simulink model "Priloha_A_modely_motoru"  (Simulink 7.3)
settings: Solver=ode23tb  StartTime=0.0  StopTime=0.5  RelTol=1e-3
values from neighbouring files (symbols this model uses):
  ILi = [0 Imax]    [Priloha_B_motor1_parametry.m]    (also in Priloha_C_motor2_parametry.m)
  Im = Psim / Ldi(1)    [Priloha_B_motor1_parametry.m]    (also in Priloha_C_motor2_parametry.m)
  Imax = 8    [Priloha_B_motor1_parametry.m]    (also in Priloha_C_motor2_parametry.m)
  J = 7e-3    (= 0.007)    [Priloha_B_motor1_parametry.m]    (also in Priloha_C_motor2_parametry.m)
  Ld = 22.5e-3    (= 0.0225)    [Priloha_B_motor1_parametry.m]    (also in Priloha_C_motor2_parametry.m)
  Ldi = [Ldi Ldi]    [Priloha_B_motor1_parametry.m]    (also in Priloha_C_motor2_parametry.m)
  Lq = 54e-3    (= 0.054)    [Priloha_B_motor1_parametry.m]    (also in Priloha_C_motor2_parametry.m)
  Lqi = [Lqi Lqi]    [Priloha_B_motor1_parametry.m]    (also in Priloha_C_motor2_parametry.m)
  p = 3    [Priloha_B_motor1_parametry.m]    (also in Priloha_C_motor2_parametry.m)
  Psim = 238.2e-3    (= 0.2382)    [Priloha_B_motor1_parametry.m]    (also in Priloha_C_motor2_parametry.m = 0.181)
  Rs = 3.95    [Priloha_B_motor1_parametry.m]    (also in Priloha_C_motor2_parametry.m)

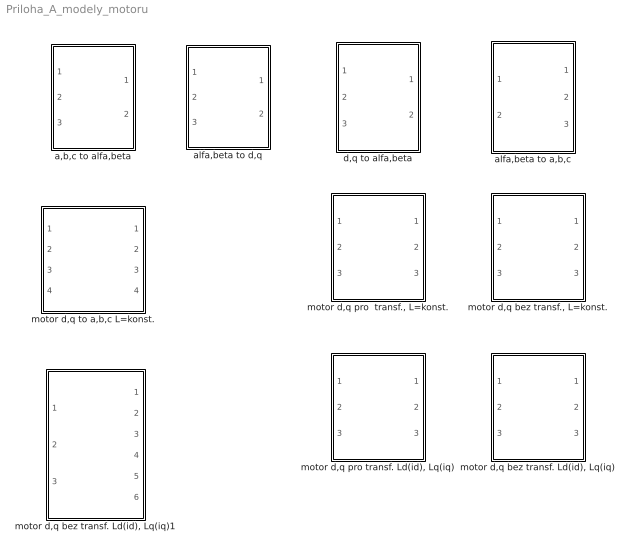
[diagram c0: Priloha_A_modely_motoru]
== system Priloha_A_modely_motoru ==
  a,b,c to alfa,beta : Subsystem
  alfa,beta to a,b,c : Subsystem
  alfa,beta to d,q : Subsystem
  d,q to alfa,beta : Subsystem
  "motor d,q bez transf., L=konst." : Subsystem
  "motor d,q bez transf. Ld(id), Lq(iq)" : Subsystem
  "motor d,q bez transf. Ld(id), Lq(iq)1" : Subsystem
  "motor d,q pro  transf., L=konst." : Subsystem
  "motor d,q pro transf. Ld(id), Lq(iq)" : Subsystem
  motor d,q to a,b,c L=konst. : Subsystem

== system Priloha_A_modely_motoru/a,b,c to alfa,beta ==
  note: transformace a, b, c do alfa, beta
  a : Inport  OutDataType=fixdt(1, 16)  OutScaling=2^0
  b : Inport  Port=2  OutDataType=fixdt(1, 16)  OutScaling=2^0
  c : Inport  Port=3  OutDataType=fixdt(1, 16)  OutScaling=2^0
  Add3 : Sum  Inputs=+-  OutDataType=fixdt(1, 16)  OutScaling=2^-10
  Gain6 : Gain  Gain=1/(sqrt(3))  ParameterDataType=fixdt(1, 16)  ParameterScaling=2^0  OutDataType=fixdt(1, 16)  OutScaling=2^0
  alfa : Outport  OutDataType=fixdt(1, 16)  OutScaling=2^0
  beta : Outport  Port=2  OutDataType=fixdt(1, 16)  OutScaling=2^0
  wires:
  a/1 -> alfa/1
  Gain6/1 -> beta/1
  Add3/1 -> Gain6/1
  b/1 -> Add3/1
  c/1 -> Add3/2

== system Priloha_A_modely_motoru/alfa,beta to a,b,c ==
  note: transformace alfa, beta do a, b, c
  alfa : Inport  OutDataType=fixdt(1, 16)  OutScaling=2^0
  beta : Inport  Port=2  OutDataType=fixdt(1, 16)  OutScaling=2^0
  Add1 : Sum  Inputs=--  OutDataType=fixdt(1, 16)  OutScaling=2^-10
  Add5 : Sum  Inputs=-+  OutDataType=fixdt(1, 16)  OutScaling=2^-10
  Gain1 : Gain  Gain=1/2  ParameterDataType=fixdt(1, 16)  ParameterScaling=2^0  OutDataType=fixdt(1, 16)  OutScaling=2^0
  Gain2 : Gain  Gain=sqrt(3)/2  ParameterDataType=fixdt(1, 16)  ParameterScaling=2^0  OutDataType=fixdt(1, 16)  OutScaling=2^0
  a : Outport  OutDataType=fixdt(1, 16)  OutScaling=2^0
  b : Outport  Port=2  OutDataType=fixdt(1, 16)  OutScaling=2^0
  c : Outport  Port=3  OutDataType=fixdt(1, 16)  OutScaling=2^0
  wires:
  alfa/1 -> a/1, Gain1/1
  Gain1/1 -> Add5/1, Add1/1
  Add5/1 -> b/1
  beta/1 -> Gain2/1
  Add1/1 -> c/1
  Gain2/1 -> Add5/2, Add1/2

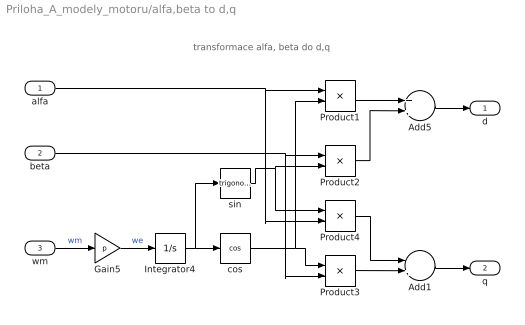
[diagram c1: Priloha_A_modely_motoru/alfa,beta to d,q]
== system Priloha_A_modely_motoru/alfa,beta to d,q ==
  note: transformace alfa, beta do d,q
  alfa : Inport  OutDataType=fixdt(1, 16)  OutScaling=2^0
  beta : Inport  Port=2  OutDataType=fixdt(1, 16)  OutScaling=2^0
  wm : Inport  Port=3  OutDataType=fixdt(1, 16)  OutScaling=2^0
  Add1 : Sum  Inputs=-+  OutDataType=fixdt(1, 16)  OutScaling=2^-10
  Add5 : Sum  OutDataType=fixdt(1, 16)  OutScaling=2^-10
  Gain5 : Gain  Gain=p  ParameterDataType=fixdt(1, 16)  ParameterScaling=2^0  OutDataType=fixdt(1, 16)  OutScaling=2^0
  Integrator4 : Integrator
  Product{1..4} (4 alike) : Product  OutDataType=fixdt(1, 16)  OutScaling=2^0
  cos : Trigonometry  Operator=cos  OutputSignalType=real
  sin : Trigonometry  OutputSignalType=real
  d : Outport  OutDataType=fixdt(1, 16)  OutScaling=2^0
  q : Outport  Port=2  OutDataType=fixdt(1, 16)  OutScaling=2^0
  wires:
  cos/1 -> Product1/2, Product3/1
  sin/1 -> Product4/1, Product2/2
  Integrator4/1 -> sin/1, cos/1
  Gain5/1 -> Integrator4/1  "we"
  wm/1 -> Gain5/1  "wm"
  Add1/1 -> q/1
  Product2/1 -> Add5/2
  beta/1 -> Product3/2, Product2/1
  alfa/1 -> Product4/2, Product1/1
  Product1/1 -> Add5/1
  Add5/1 -> d/1
  Product4/1 -> Add1/1
  Product3/1 -> Add1/2

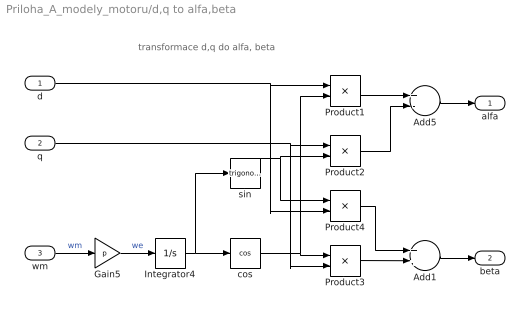
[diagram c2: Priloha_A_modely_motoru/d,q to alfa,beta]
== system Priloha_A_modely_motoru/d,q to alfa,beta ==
  note: transformace d,q do alfa, beta
  d : Inport  OutDataType=fixdt(1, 16)  OutScaling=2^0
  q : Inport  Port=2  OutDataType=fixdt(1, 16)  OutScaling=2^0
  wm : Inport  Port=3  OutDataType=fixdt(1, 16)  OutScaling=2^0
  Add1 : Sum  OutDataType=fixdt(1, 16)  OutScaling=2^-10
  Add5 : Sum  Inputs=+-  OutDataType=fixdt(1, 16)  OutScaling=2^-10
  Gain5 : Gain  Gain=p  ParameterDataType=fixdt(1, 16)  ParameterScaling=2^0  OutDataType=fixdt(1, 16)  OutScaling=2^0
  Integrator4 : Integrator
  Product{1..4} (4 alike) : Product  OutDataType=fixdt(1, 16)  OutScaling=2^0
  cos : Trigonometry  Operator=cos
  sin : Trigonometry
  alfa : Outport  OutDataType=fixdt(1, 16)  OutScaling=2^0
  beta : Outport  Port=2  OutDataType=fixdt(1, 16)  OutScaling=2^0
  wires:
  Add5/1 -> alfa/1
  Product1/1 -> Add5/1
  d/1 -> Product4/2, Product1/1
  q/1 -> Product3/2, Product2/1
  Product2/1 -> Add5/2
  Add1/1 -> beta/1
  wm/1 -> Gain5/1  "wm"
  Gain5/1 -> Integrator4/1  "we"
  Integrator4/1 -> sin/1, cos/1
  sin/1 -> Product4/1, Product2/2
  cos/1 -> Product1/2, Product3/1
  Product4/1 -> Add1/1
  Product3/1 -> Add1/2

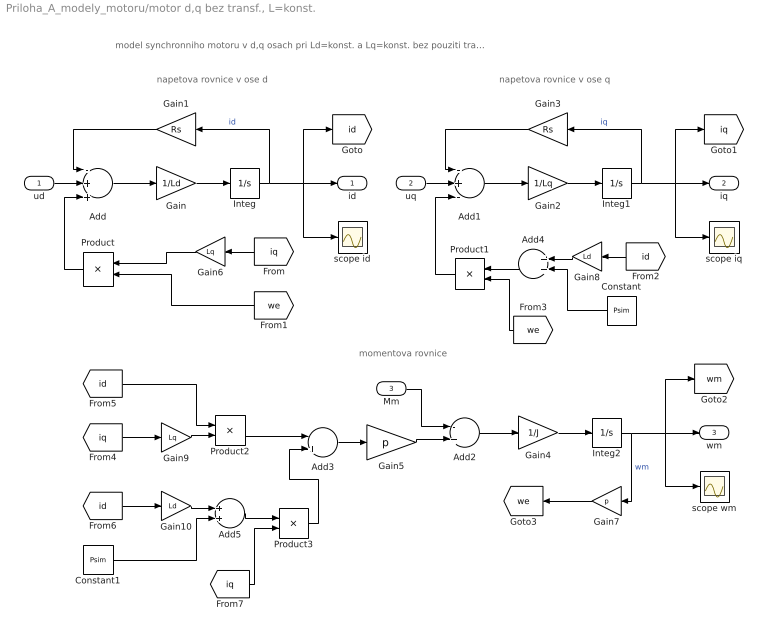
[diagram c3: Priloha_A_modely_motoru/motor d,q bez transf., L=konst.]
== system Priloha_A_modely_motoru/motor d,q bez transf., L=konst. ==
  note: momentova rovnice
  note: napetova rovnice v ose q
  note: napetova rovnice v ose d
  note: model synchronniho motoru v d,q osach pri Ld=konst. a Lq=konst. bez pouziti transformace (v momentove rovnici neni koeficient 3/2)
  ud : Inport  OutDataType=fixdt(1, 16)  OutScaling=2^0
  uq : Inport  Port=2  OutDataType=fixdt(1, 16)  OutScaling=2^0
  Mm : Inport  Port=3  OutDataType=fixdt(1, 16)  OutScaling=2^0
  Add : Sum  Inputs=-++  OutDataType=fixdt(1, 16)  OutScaling=2^-10
  Add1 : Sum  Inputs=-+-  OutDataType=fixdt(1, 16)  OutScaling=2^-10
  Add2 : Sum  Inputs=-+  OutDataType=fixdt(1, 16)  OutScaling=2^-10
  Add3 : Sum  Inputs=-+  OutDataType=fixdt(1, 16)  OutScaling=2^-10
  Add4 : Sum  OutDataType=fixdt(1, 16)  OutScaling=2^-10
  Add5 : Sum  OutDataType=fixdt(1, 16)  OutScaling=2^-10
  Constant : Constant  Value=Psim  OutDataType=fixdt(1, 16)  OutScaling=2^0
  Constant1 : Constant  Value=Psim  OutDataType=fixdt(1, 16)  OutScaling=2^0
  Gain : Gain  Gain=1/Ld  ParameterDataType=fixdt(1, 16)  ParameterScaling=2^0  OutDataType=fixdt(1, 16)  OutScaling=2^0
  Gain1 : Gain  Gain=Rs  ParameterDataType=fixdt(1, 16)  ParameterScaling=2^0  OutDataType=fixdt(1, 16)  OutScaling=2^0
  Gain10 : Gain  Gain=Ld  ParameterDataType=fixdt(1, 16)  ParameterScaling=2^0  OutDataType=fixdt(1, 16)  OutScaling=2^0
  Gain2 : Gain  Gain=1/Lq  ParameterDataType=fixdt(1, 16)  ParameterScaling=2^0  OutDataType=fixdt(1, 16)  OutScaling=2^0
  Gain3 : Gain  Gain=Rs  ParameterDataType=fixdt(1, 16)  ParameterScaling=2^0  OutDataType=fixdt(1, 16)  OutScaling=2^0
  Gain4 : Gain  Gain=1/J  ParameterDataType=fixdt(1, 16)  ParameterScaling=2^0  OutDataType=fixdt(1, 16)  OutScaling=2^0
  Gain5 : Gain  Gain=p  ParameterDataType=fixdt(1, 16)  ParameterScaling=2^0  OutDataType=fixdt(1, 16)  OutScaling=2^0
  Gain6 : Gain  Gain=Lq  ParameterDataType=fixdt(1, 16)  ParameterScaling=2^0  OutDataType=fixdt(1, 16)  OutScaling=2^0
  Gain7 : Gain  Gain=p  ParameterDataType=fixdt(1, 16)  ParameterScaling=2^0  OutDataType=fixdt(1, 16)  OutScaling=2^0
  Gain8 : Gain  Gain=Ld  ParameterDataType=fixdt(1, 16)  ParameterScaling=2^0  OutDataType=fixdt(1, 16)  OutScaling=2^0
  Gain9 : Gain  Gain=Lq  ParameterDataType=fixdt(1, 16)  ParameterScaling=2^0  OutDataType=fixdt(1, 16)  OutScaling=2^0
  Integ : Integrator
  Integ1 : Integrator
  Integ2 : Integrator
  Product{,1..3} (4 alike) : Product  OutDataType=fixdt(1, 16)  OutScaling=2^0
  scope id : Scope
  scope iq : Scope
  scope wm : Scope
  id : Outport  OutDataType=fixdt(1, 16)  OutScaling=2^0
  iq : Outport  Port=2  OutDataType=fixdt(1, 16)  OutScaling=2^0
  wm : Outport  Port=3  OutDataType=fixdt(1, 16)  OutScaling=2^0
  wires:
  [we] -> Product/2
  Gain6/1 -> Product/1
  [iq] -> Gain6/1
  Constant/1 -> Add4/2
  Product/1 -> Add/3
  [we] -> Product1/2
  Product1/1 -> Add1/3
  Product3/1 -> Add3/2
  [iq] -> Product3/2
  Constant1/1 -> Add5/2
  Add5/1 -> Product3/1
  Gain10/1 -> Add5/1
  [id] -> Gain10/1
  Product2/1 -> Add3/1
  Gain9/1 -> Product2/2
  [id] -> Product2/1
  [iq] -> Gain9/1
  Add4/1 -> Product1/1
  Gain8/1 -> Add4/1
  [id] -> Gain8/1
  Gain7/1 -> [we]
  Add3/1 -> Gain5/1
  Mm/1 -> Add2/1
  Gain5/1 -> Add2/2
  Add2/1 -> Gain4/1
  Gain4/1 -> Integ2/1
  Integ2/1 -> Gain7/1, [wm], scope wm/1, wm/1  "wm"
  uq/1 -> Add1/2
  Gain3/1 -> Add1/1
  Add1/1 -> Gain2/1
  Gain2/1 -> Integ1/1
  Integ1/1 -> [iq], iq/1, scope iq/1, Gain3/1  "iq"
  ud/1 -> Add/2
  Gain1/1 -> Add/1
  Add/1 -> Gain/1
  Gain/1 -> Integ/1
  Integ/1 -> Gain1/1, [id], scope id/1, id/1  "id"

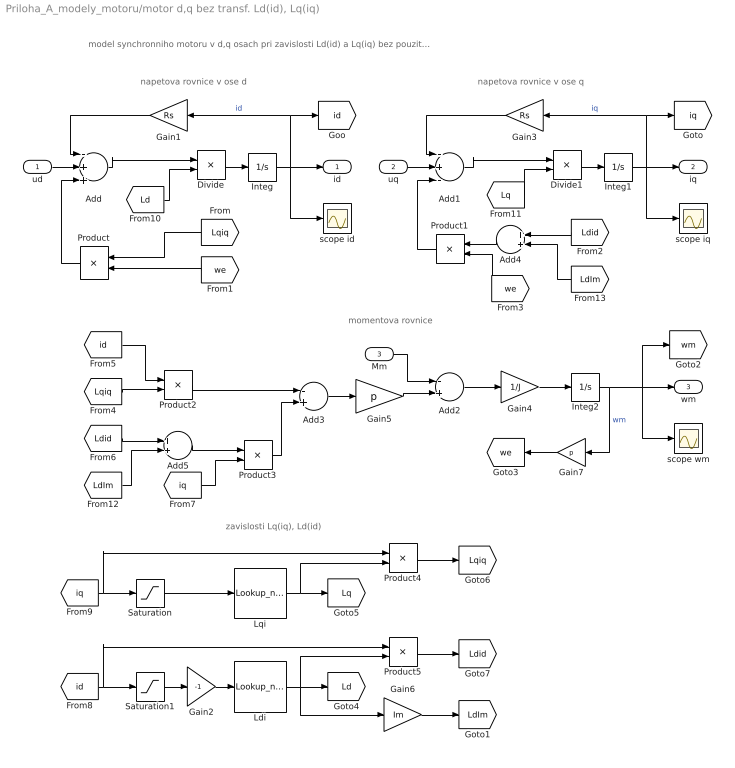
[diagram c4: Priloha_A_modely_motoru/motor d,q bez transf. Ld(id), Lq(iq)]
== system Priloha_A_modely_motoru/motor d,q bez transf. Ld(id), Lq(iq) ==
  note: zavislosti Lq(iq), Ld(id)
  note: momentova rovnice
  note: napetova rovnice v ose q
  note: napetova rovnice v ose d
  note: model synchronniho motoru v d,q osach pri zavislosti Ld(id) a Lq(iq) bez pouziti transformace (v momentove rovnici neni koeficient 3/2)
  ud : Inport  OutDataType=fixdt(1, 16)  OutScaling=2^0
  uq : Inport  Port=2  OutDataType=fixdt(1, 16)  OutScaling=2^0
  Mm : Inport  Port=3  OutDataType=fixdt(1, 16)  OutScaling=2^0
  Add : Sum  Inputs=-++  OutDataType=fixdt(1, 16)  OutScaling=2^-10
  Add1 : Sum  Inputs=-+-  OutDataType=fixdt(1, 16)  OutScaling=2^-10
  Add2 : Sum  Inputs=-+  OutDataType=fixdt(1, 16)  OutScaling=2^-10
  Add3 : Sum  Inputs=-+  OutDataType=fixdt(1, 16)  OutScaling=2^-10
  Add4 : Sum  OutDataType=fixdt(1, 16)  OutScaling=2^-10
  Add5 : Sum  OutDataType=fixdt(1, 16)  OutScaling=2^-10
  Divide : Product  Inputs=*/  OutDataType=fixdt(1, 16)  OutScaling=2^-10
  Divide1 : Product  Inputs=*/  OutDataType=fixdt(1, 16)  OutScaling=2^-10
  Gain1 : Gain  Gain=Rs  ParameterDataType=fixdt(1, 16)  ParameterScaling=2^0  OutDataType=fixdt(1, 16)  OutScaling=2^0
  Gain2 : Gain  Gain=-1  ParameterDataType=fixdt(1, 16)  ParameterScaling=2^0  OutDataType=fixdt(1, 16)  OutScaling=2^0
  Gain3 : Gain  Gain=Rs  ParameterDataType=fixdt(1, 16)  ParameterScaling=2^0  OutDataType=fixdt(1, 16)  OutScaling=2^0
  Gain4 : Gain  Gain=1/J  ParameterDataType=fixdt(1, 16)  ParameterScaling=2^0  OutDataType=fixdt(1, 16)  OutScaling=2^0
  Gain5 : Gain  Gain=p  ParameterDataType=fixdt(1, 16)  ParameterScaling=2^0  OutDataType=fixdt(1, 16)  OutScaling=2^0
  Gain6 : Gain  Gain=Im  ParameterDataType=fixdt(1, 16)  ParameterScaling=2^0  OutDataType=fixdt(1, 16)  OutScaling=2^0
  Gain7 : Gain  Gain=p  ParameterDataType=fixdt(1, 16)  ParameterScaling=2^0  OutDataType=fixdt(1, 16)  OutScaling=2^0
  Integ : Integrator
  Integ1 : Integrator
  Integ2 : Integrator
  Ldi : Lookup_n-D  NumberOfTableDimensions=1  BreakpointsForDimension1=[ILi]  Table=[Ldi]
  Lqi : Lookup_n-D  NumberOfTableDimensions=1  BreakpointsForDimension1=[ILi]  Table=[Lqi]
  Product{,1..5} (6 alike) : Product  OutDataType=fixdt(1, 16)  OutScaling=2^0
  Saturation : Saturate  UpperLimit=Imax  LowerLimit=ILi(1)  OutDataType=fixdt(1, 16)  OutScaling=2^0
  Saturation1 : Saturate  UpperLimit=ILi(1)  LowerLimit=-Imax  OutDataType=fixdt(1, 16)  OutScaling=2^0
  scope id : Scope
  scope iq : Scope
  scope wm : Scope
  id : Outport  OutDataType=fixdt(1, 16)  OutScaling=2^0
  iq : Outport  Port=2  OutDataType=fixdt(1, 16)  OutScaling=2^0
  wm : Outport  Port=3  OutDataType=fixdt(1, 16)  OutScaling=2^0
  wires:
  [LdIm] -> Add4/2
  [LdIm] -> Add5/2
  Gain6/1 -> [LdIm]
  Gain2/1 -> Ldi/1
  [Lq] -> Divide1/2
  Add1/1 -> Divide1/1
  [Lqiq] -> Product/1
  Divide1/1 -> Integ1/1
  [Ld] -> Divide/2
  Add/1 -> Divide/1
  Divide/1 -> Integ/1
  Product5/1 -> [Ldid]
  Product4/1 -> [Lqiq]
  Ldi/1 -> Gain6/1, Product5/2, [Ld]
  [id] -> Product5/1, Saturation1/1
  Lqi/1 -> Product4/2, [Lq]
  [iq] -> Product4/1, Saturation/1
  Saturation1/1 -> Gain2/1
  Saturation/1 -> Lqi/1
  [we] -> Product/2
  Product/1 -> Add/3
  [we] -> Product1/2
  Product1/1 -> Add1/3
  Product3/1 -> Add3/2
  [iq] -> Product3/2
  Add5/1 -> Product3/1
  [Ldid] -> Add5/1
  Product2/1 -> Add3/1
  [id] -> Product2/1
  [Lqiq] -> Product2/2
  Add4/1 -> Product1/1
  [Ldid] -> Add4/1
  Gain7/1 -> [we]
  Add3/1 -> Gain5/1
  Mm/1 -> Add2/1
  Gain5/1 -> Add2/2
  Add2/1 -> Gain4/1
  Gain4/1 -> Integ2/1
  Integ2/1 -> Gain7/1, [wm], scope wm/1, wm/1  "wm"
  uq/1 -> Add1/2
  Gain3/1 -> Add1/1
  Integ1/1 -> Gain3/1, [iq], iq/1, scope iq/1  "iq"
  ud/1 -> Add/2
  Gain1/1 -> Add/1
  Integ/1 -> Gain1/1, [id], scope id/1, id/1  "id"

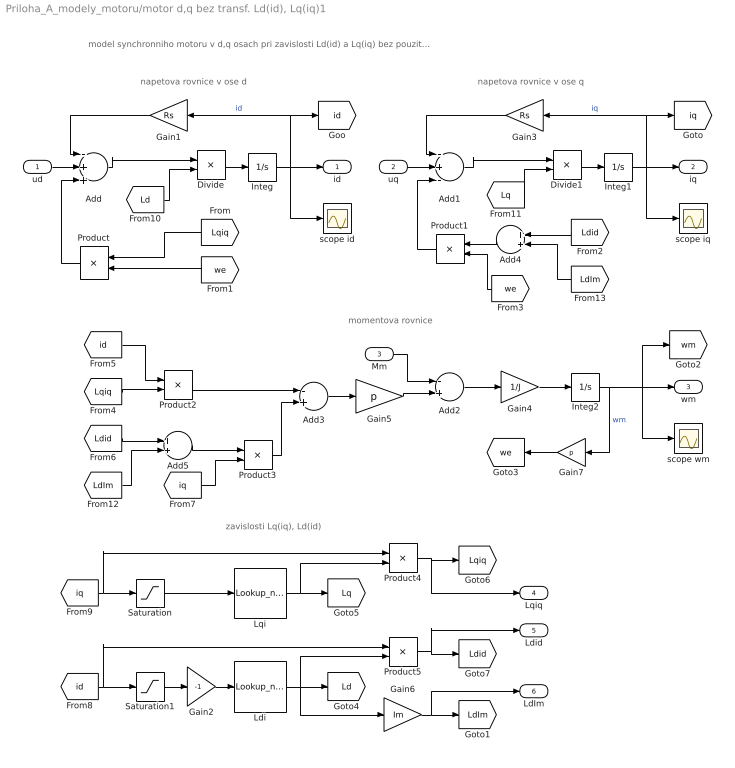
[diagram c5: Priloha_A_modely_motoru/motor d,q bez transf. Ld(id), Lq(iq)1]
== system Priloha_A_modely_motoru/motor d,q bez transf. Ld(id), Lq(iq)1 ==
  note: model synchronniho motoru v d,q osach pri zavislosti Ld(id) a Lq(iq) bez pouziti transformace (v momentove rovnici neni koeficient 3/2)
  note: napetova rovnice v ose d
  note: napetova rovnice v ose q
  note: momentova rovnice
  note: zavislosti Lq(iq), Ld(id)
  ud : Inport  OutDataType=fixdt(1, 16)  OutScaling=2^0
  uq : Inport  Port=2  OutDataType=fixdt(1, 16)  OutScaling=2^0
  Mm : Inport  Port=3  OutDataType=fixdt(1, 16)  OutScaling=2^0
  Add : Sum  Inputs=-++  OutDataType=fixdt(1, 16)  OutScaling=2^-10
  Add1 : Sum  Inputs=-+-  OutDataType=fixdt(1, 16)  OutScaling=2^-10
  Add2 : Sum  Inputs=-+  OutDataType=fixdt(1, 16)  OutScaling=2^-10
  Add3 : Sum  Inputs=-+  OutDataType=fixdt(1, 16)  OutScaling=2^-10
  Add4 : Sum  OutDataType=fixdt(1, 16)  OutScaling=2^-10
  Add5 : Sum  OutDataType=fixdt(1, 16)  OutScaling=2^-10
  Divide : Product  Inputs=*/  OutDataType=fixdt(1, 16)  OutScaling=2^-10
  Divide1 : Product  Inputs=*/  OutDataType=fixdt(1, 16)  OutScaling=2^-10
  Gain1 : Gain  Gain=Rs  ParameterDataType=fixdt(1, 16)  ParameterScaling=2^0  OutDataType=fixdt(1, 16)  OutScaling=2^0
  Gain2 : Gain  Gain=-1  ParameterDataType=fixdt(1, 16)  ParameterScaling=2^0  OutDataType=fixdt(1, 16)  OutScaling=2^0
  Gain3 : Gain  Gain=Rs  ParameterDataType=fixdt(1, 16)  ParameterScaling=2^0  OutDataType=fixdt(1, 16)  OutScaling=2^0
  Gain4 : Gain  Gain=1/J  ParameterDataType=fixdt(1, 16)  ParameterScaling=2^0  OutDataType=fixdt(1, 16)  OutScaling=2^0
  Gain5 : Gain  Gain=p  ParameterDataType=fixdt(1, 16)  ParameterScaling=2^0  OutDataType=fixdt(1, 16)  OutScaling=2^0
  Gain6 : Gain  Gain=Im  ParameterDataType=fixdt(1, 16)  ParameterScaling=2^0  OutDataType=fixdt(1, 16)  OutScaling=2^0
  Gain7 : Gain  Gain=p  ParameterDataType=fixdt(1, 16)  ParameterScaling=2^0  OutDataType=fixdt(1, 16)  OutScaling=2^0
  Integ : Integrator
  Integ1 : Integrator
  Integ2 : Integrator
  Ldi : Lookup_n-D  NumberOfTableDimensions=1  BreakpointsForDimension1=[ILi]  Table=[Ldi]
  Lqi : Lookup_n-D  NumberOfTableDimensions=1  BreakpointsForDimension1=[ILi]  Table=[Lqi]
  Product{,1..5} (6 alike) : Product  OutDataType=fixdt(1, 16)  OutScaling=2^0
  Saturation : Saturate  UpperLimit=Imax  LowerLimit=ILi(1)  OutDataType=fixdt(1, 16)  OutScaling=2^0
  Saturation1 : Saturate  UpperLimit=ILi(1)  LowerLimit=-Imax  OutDataType=fixdt(1, 16)  OutScaling=2^0
  scope id : Scope
  scope iq : Scope
  scope wm : Scope
  id : Outport  OutDataType=fixdt(1, 16)  OutScaling=2^0
  iq : Outport  Port=2  OutDataType=fixdt(1, 16)  OutScaling=2^0
  wm : Outport  Port=3  OutDataType=fixdt(1, 16)  OutScaling=2^0
  Lqiq : Outport  Port=4  OutDataType=fixdt(1, 16)  OutScaling=2^0
  Ldid : Outport  Port=5  OutDataType=fixdt(1, 16)  OutScaling=2^0
  LdIm : Outport  Port=6  OutDataType=fixdt(1, 16)  OutScaling=2^0
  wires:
  Integ/1 -> id/1, scope id/1, [id], Gain1/1  "id"
  Gain1/1 -> Add/1
  ud/1 -> Add/2
  Integ1/1 -> scope iq/1, iq/1, [iq], Gain3/1  "iq"
  Gain3/1 -> Add1/1
  uq/1 -> Add1/2
  Integ2/1 -> wm/1, scope wm/1, [wm], Gain7/1  "wm"
  Gain4/1 -> Integ2/1
  Add2/1 -> Gain4/1
  Gain5/1 -> Add2/2
  Mm/1 -> Add2/1
  Add3/1 -> Gain5/1
  Gain7/1 -> [we]
  [Ldid] -> Add4/1
  Add4/1 -> Product1/1
  [Lqiq] -> Product2/2
  [id] -> Product2/1
  Product2/1 -> Add3/1
  [Ldid] -> Add5/1
  Add5/1 -> Product3/1
  [iq] -> Product3/2
  Product3/1 -> Add3/2
  Product1/1 -> Add1/3
  Product/1 -> Add/3
  Saturation/1 -> Lqi/1
  Saturation1/1 -> Gain2/1
  [iq] -> Saturation/1, Product4/1
  Lqi/1 -> [Lq], Product4/2
  [id] -> Saturation1/1, Product5/1
  Ldi/1 -> [Ld], Product5/2, Gain6/1
  Product4/1 -> [Lqiq], Lqiq/1
  Product5/1 -> [Ldid], Ldid/1
  Divide/1 -> Integ/1
  Add/1 -> Divide/1
  [Ld] -> Divide/2
  Divide1/1 -> Integ1/1
  [Lqiq] -> Product/1
  Add1/1 -> Divide1/1
  [Lq] -> Divide1/2
  Gain2/1 -> Ldi/1
  Gain6/1 -> [LdIm], LdIm/1
  [LdIm] -> Add5/2
  [LdIm] -> Add4/2
  [we] -> Product1/2
  [we] -> Product/2

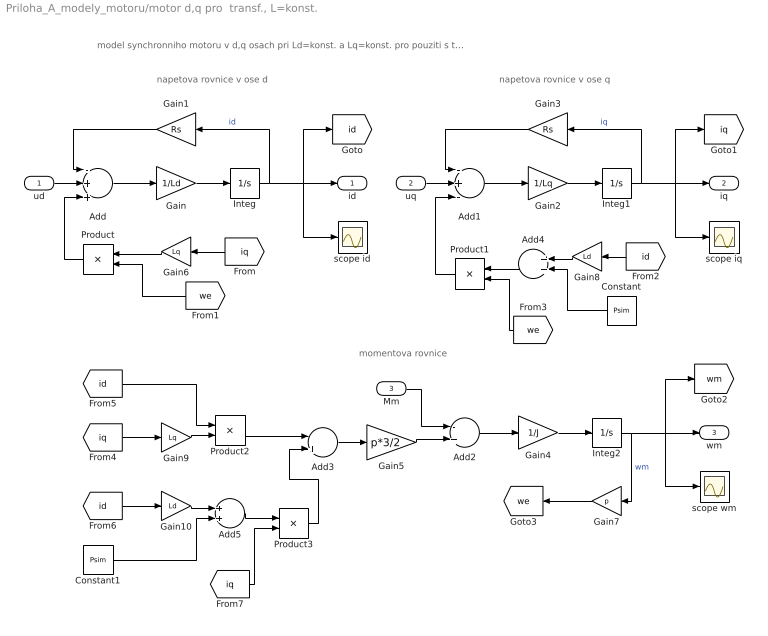
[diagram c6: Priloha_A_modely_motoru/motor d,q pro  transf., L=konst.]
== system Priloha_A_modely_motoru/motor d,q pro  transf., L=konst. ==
  note: momentova rovnice
  note: napetova rovnice v ose q
  note: napetova rovnice v ose d
  note: model synchronniho motoru v d,q osach pri Ld=konst. a Lq=konst. pro pouziti s transformaci (v momentove rovnici je koeficient 3/2)
  ud : Inport  OutDataType=fixdt(1, 16)  OutScaling=2^0
  uq : Inport  Port=2  OutDataType=fixdt(1, 16)  OutScaling=2^0
  Mm : Inport  Port=3  OutDataType=fixdt(1, 16)  OutScaling=2^0
  Add : Sum  Inputs=-++  OutDataType=fixdt(1, 16)  OutScaling=2^-10
  Add1 : Sum  Inputs=-+-  OutDataType=fixdt(1, 16)  OutScaling=2^-10
  Add2 : Sum  Inputs=-+  OutDataType=fixdt(1, 16)  OutScaling=2^-10
  Add3 : Sum  Inputs=-+  OutDataType=fixdt(1, 16)  OutScaling=2^-10
  Add4 : Sum  OutDataType=fixdt(1, 16)  OutScaling=2^-10
  Add5 : Sum  OutDataType=fixdt(1, 16)  OutScaling=2^-10
  Constant : Constant  Value=Psim  OutDataType=fixdt(1, 16)  OutScaling=2^0
  Constant1 : Constant  Value=Psim  OutDataType=fixdt(1, 16)  OutScaling=2^0
  Gain : Gain  Gain=1/Ld  ParameterDataType=fixdt(1, 16)  ParameterScaling=2^0  OutDataType=fixdt(1, 16)  OutScaling=2^0
  Gain1 : Gain  Gain=Rs  ParameterDataType=fixdt(1, 16)  ParameterScaling=2^0  OutDataType=fixdt(1, 16)  OutScaling=2^0
  Gain10 : Gain  Gain=Ld  ParameterDataType=fixdt(1, 16)  ParameterScaling=2^0  OutDataType=fixdt(1, 16)  OutScaling=2^0
  Gain2 : Gain  Gain=1/Lq  ParameterDataType=fixdt(1, 16)  ParameterScaling=2^0  OutDataType=fixdt(1, 16)  OutScaling=2^0
  Gain3 : Gain  Gain=Rs  ParameterDataType=fixdt(1, 16)  ParameterScaling=2^0  OutDataType=fixdt(1, 16)  OutScaling=2^0
  Gain4 : Gain  Gain=1/J  ParameterDataType=fixdt(1, 16)  ParameterScaling=2^0  OutDataType=fixdt(1, 16)  OutScaling=2^0
  Gain5 : Gain  Gain=p*3/2  ParameterDataType=fixdt(1, 16)  ParameterScaling=2^0  OutDataType=fixdt(1, 16)  OutScaling=2^0
  Gain6 : Gain  Gain=Lq  ParameterDataType=fixdt(1, 16)  ParameterScaling=2^0  OutDataType=fixdt(1, 16)  OutScaling=2^0
  Gain7 : Gain  Gain=p  ParameterDataType=fixdt(1, 16)  ParameterScaling=2^0  OutDataType=fixdt(1, 16)  OutScaling=2^0
  Gain8 : Gain  Gain=Ld  ParameterDataType=fixdt(1, 16)  ParameterScaling=2^0  OutDataType=fixdt(1, 16)  OutScaling=2^0
  Gain9 : Gain  Gain=Lq  ParameterDataType=fixdt(1, 16)  ParameterScaling=2^0  OutDataType=fixdt(1, 16)  OutScaling=2^0
  Integ : Integrator
  Integ1 : Integrator
  Integ2 : Integrator
  Product{,1..3} (4 alike) : Product  OutDataType=fixdt(1, 16)  OutScaling=2^0
  scope id : Scope
  scope iq : Scope
  scope wm : Scope
  id : Outport  OutDataType=fixdt(1, 16)  OutScaling=2^0
  iq : Outport  Port=2  OutDataType=fixdt(1, 16)  OutScaling=2^0
  wm : Outport  Port=3  OutDataType=fixdt(1, 16)  OutScaling=2^0
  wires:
  [we] -> Product/2
  Constant/1 -> Add4/2
  Product/1 -> Add/3
  [we] -> Product1/2
  Product1/1 -> Add1/3
  Product3/1 -> Add3/2
  [iq] -> Product3/2
  Constant1/1 -> Add5/2
  Add5/1 -> Product3/1
  Gain10/1 -> Add5/1
  [id] -> Gain10/1
  Product2/1 -> Add3/1
  Gain9/1 -> Product2/2
  [id] -> Product2/1
  [iq] -> Gain9/1
  Add4/1 -> Product1/1
  Gain8/1 -> Add4/1
  [id] -> Gain8/1
  Gain7/1 -> [we]
  Gain6/1 -> Product/1
  [iq] -> Gain6/1
  Add3/1 -> Gain5/1
  Mm/1 -> Add2/1
  Gain5/1 -> Add2/2
  Add2/1 -> Gain4/1
  Gain4/1 -> Integ2/1
  Integ2/1 -> Gain7/1, [wm], scope wm/1, wm/1  "wm"
  uq/1 -> Add1/2
  Gain3/1 -> Add1/1
  Add1/1 -> Gain2/1
  Gain2/1 -> Integ1/1
  Integ1/1 -> [iq], iq/1, scope iq/1, Gain3/1  "iq"
  ud/1 -> Add/2
  Gain1/1 -> Add/1
  Add/1 -> Gain/1
  Gain/1 -> Integ/1
  Integ/1 -> Gain1/1, [id], scope id/1, id/1  "id"

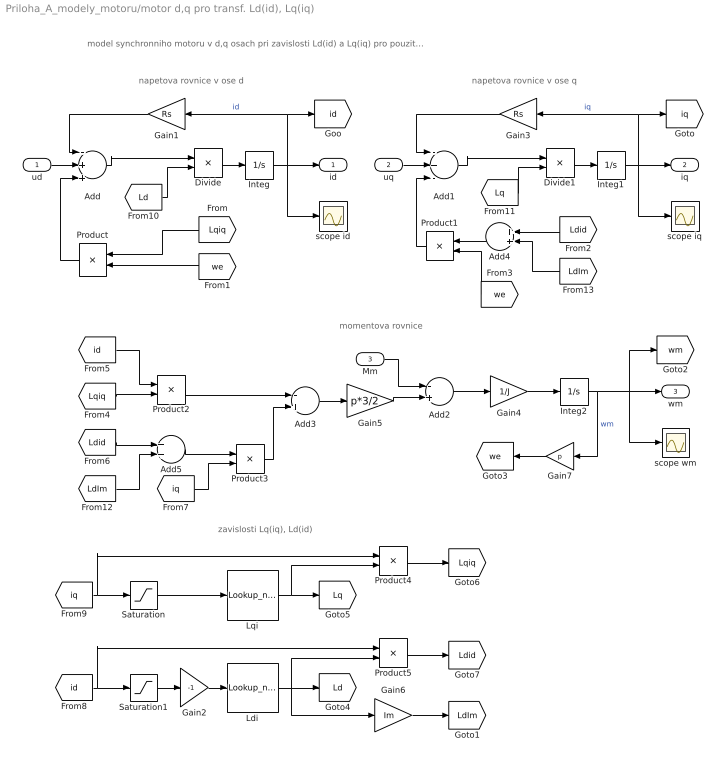
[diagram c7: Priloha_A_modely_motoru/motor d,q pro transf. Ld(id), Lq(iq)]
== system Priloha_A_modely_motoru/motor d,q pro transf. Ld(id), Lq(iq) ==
  note: model synchronniho motoru v d,q osach pri zavislosti Ld(id) a Lq(iq) pro pouziti s transformaci (v momentove rovnici je koeficient 3/2)
  note: napetova rovnice v ose d
  note: napetova rovnice v ose q
  note: momentova rovnice
  note: zavislosti Lq(iq), Ld(id)
  ud : Inport  OutDataType=fixdt(1, 16)  OutScaling=2^0
  uq : Inport  Port=2  OutDataType=fixdt(1, 16)  OutScaling=2^0
  Mm : Inport  Port=3  OutDataType=fixdt(1, 16)  OutScaling=2^0
  Add : Sum  Inputs=-++  OutDataType=fixdt(1, 16)  OutScaling=2^-10
  Add1 : Sum  Inputs=-+-  OutDataType=fixdt(1, 16)  OutScaling=2^-10
  Add2 : Sum  Inputs=-+  OutDataType=fixdt(1, 16)  OutScaling=2^-10
  Add3 : Sum  Inputs=-+  OutDataType=fixdt(1, 16)  OutScaling=2^-10
  Add4 : Sum  OutDataType=fixdt(1, 16)  OutScaling=2^-10
  Add5 : Sum  OutDataType=fixdt(1, 16)  OutScaling=2^-10
  Divide : Product  Inputs=*/  OutDataType=fixdt(1, 16)  OutScaling=2^-10
  Divide1 : Product  Inputs=*/  OutDataType=fixdt(1, 16)  OutScaling=2^-10
  Gain1 : Gain  Gain=Rs  ParameterDataType=fixdt(1, 16)  ParameterScaling=2^0  OutDataType=fixdt(1, 16)  OutScaling=2^0
  Gain2 : Gain  Gain=-1  ParameterDataType=fixdt(1, 16)  ParameterScaling=2^0  OutDataType=fixdt(1, 16)  OutScaling=2^0
  Gain3 : Gain  Gain=Rs  ParameterDataType=fixdt(1, 16)  ParameterScaling=2^0  OutDataType=fixdt(1, 16)  OutScaling=2^0
  Gain4 : Gain  Gain=1/J  ParameterDataType=fixdt(1, 16)  ParameterScaling=2^0  OutDataType=fixdt(1, 16)  OutScaling=2^0
  Gain5 : Gain  Gain=p*3/2  ParameterDataType=fixdt(1, 16)  ParameterScaling=2^0  OutDataType=fixdt(1, 16)  OutScaling=2^0
  Gain6 : Gain  Gain=Im  ParameterDataType=fixdt(1, 16)  ParameterScaling=2^0  OutDataType=fixdt(1, 16)  OutScaling=2^0
  Gain7 : Gain  Gain=p  ParameterDataType=fixdt(1, 16)  ParameterScaling=2^0  OutDataType=fixdt(1, 16)  OutScaling=2^0
  Integ : Integrator
  Integ1 : Integrator
  Integ2 : Integrator
  Ldi : Lookup_n-D  NumberOfTableDimensions=1  BreakpointsForDimension1=[ILi]  Table=[Ldi]
  Lqi : Lookup_n-D  NumberOfTableDimensions=1  BreakpointsForDimension1=[ILi]  Table=[Lqi]
  Product{,1..5} (6 alike) : Product  OutDataType=fixdt(1, 16)  OutScaling=2^0
  Saturation : Saturate  UpperLimit=Imax  LowerLimit=ILi(1)  OutDataType=fixdt(1, 16)  OutScaling=2^0
  Saturation1 : Saturate  UpperLimit=ILi(1)  LowerLimit=-Imax  OutDataType=fixdt(1, 16)  OutScaling=2^0
  scope id : Scope
  scope iq : Scope
  scope wm : Scope
  id : Outport  OutDataType=fixdt(1, 16)  OutScaling=2^0
  iq : Outport  Port=2  OutDataType=fixdt(1, 16)  OutScaling=2^0
  wm : Outport  Port=3  OutDataType=fixdt(1, 16)  OutScaling=2^0
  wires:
  Gain6/1 -> [LdIm]
  Integ/1 -> id/1, scope id/1, [id], Gain1/1  "id"
  Gain1/1 -> Add/1
  ud/1 -> Add/2
  Integ1/1 -> scope iq/1, iq/1, [iq], Gain3/1  "iq"
  Gain3/1 -> Add1/1
  uq/1 -> Add1/2
  Integ2/1 -> wm/1, scope wm/1, [wm], Gain7/1  "wm"
  Gain4/1 -> Integ2/1
  Add2/1 -> Gain4/1
  Gain5/1 -> Add2/2
  Mm/1 -> Add2/1
  Add3/1 -> Gain5/1
  Gain7/1 -> [we]
  [Ldid] -> Add4/1
  Add4/1 -> Product1/1
  [Lqiq] -> Product2/2
  [id] -> Product2/1
  Product2/1 -> Add3/1
  [Ldid] -> Add5/1
  Add5/1 -> Product3/1
  [LdIm] -> Add5/2
  [iq] -> Product3/2
  Product3/1 -> Add3/2
  Product1/1 -> Add1/3
  [we] -> Product1/2
  Product/1 -> Add/3
  [LdIm] -> Add4/2
  [we] -> Product/2
  Saturation/1 -> Lqi/1
  Saturation1/1 -> Gain2/1
  [iq] -> Saturation/1, Product4/1
  Lqi/1 -> [Lq], Product4/2
  [id] -> Saturation1/1, Product5/1
  Ldi/1 -> Gain6/1, [Ld], Product5/2
  Product4/1 -> [Lqiq]
  Product5/1 -> [Ldid]
  Divide/1 -> Integ/1
  Add/1 -> Divide/1
  [Ld] -> Divide/2
  Divide1/1 -> Integ1/1
  [Lqiq] -> Product/1
  Add1/1 -> Divide1/1
  [Lq] -> Divide1/2
  Gain2/1 -> Ldi/1

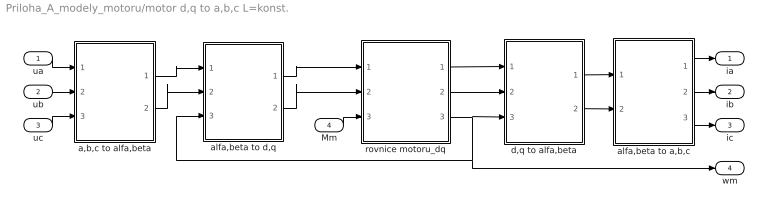
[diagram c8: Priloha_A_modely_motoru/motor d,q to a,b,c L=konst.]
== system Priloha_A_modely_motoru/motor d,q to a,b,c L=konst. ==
  ua : Inport
  ub : Inport  Port=2
  uc : Inport  Port=3
  Mm : Inport  Port=4
  a,b,c to alfa,beta : Subsystem
  alfa,beta to a,b,c : Subsystem
  alfa,beta to d,q : Subsystem
  d,q to alfa,beta : Subsystem
  rovnice motoru_dq : Subsystem
  ia : Outport
  ib : Outport  Port=2
  ic : Outport  Port=3
  wm : Outport  Port=4
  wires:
  a,b,c to alfa,beta/1(alfa) -> alfa,beta to d,q/1(alfa)
  a,b,c to alfa,beta/2(beta) -> alfa,beta to d,q/2(beta)
  rovnice motoru_dq/1(id) -> d,q to alfa,beta/1(d)
  rovnice motoru_dq/2(iq) -> d,q to alfa,beta/2(q)
  rovnice motoru_dq/3(wm) -> d,q to alfa,beta/3(wm), alfa,beta to d,q/3(wm), wm/1
  d,q to alfa,beta/1(alfa) -> alfa,beta to a,b,c/1(alfa)
  d,q to alfa,beta/2(beta) -> alfa,beta to a,b,c/2(beta)
  alfa,beta to d,q/1(d) -> rovnice motoru_dq/1(ud)
  alfa,beta to d,q/2(q) -> rovnice motoru_dq/2(uq)
  ua/1 -> a,b,c to alfa,beta/1(a)
  alfa,beta to a,b,c/1(a) -> ia/1
  ub/1 -> a,b,c to alfa,beta/2(b)
  alfa,beta to a,b,c/2(b) -> ib/1
  uc/1 -> a,b,c to alfa,beta/3(c)
  alfa,beta to a,b,c/3(c) -> ic/1
  Mm/1 -> rovnice motoru_dq/3(Mm)

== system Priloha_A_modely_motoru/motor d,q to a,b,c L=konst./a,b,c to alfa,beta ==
  note: transformace a, b, c do alfa, beta
  a : Inport  OutDataType=fixdt(1, 16)  OutScaling=2^0
  b : Inport  Port=2  OutDataType=fixdt(1, 16)  OutScaling=2^0
  c : Inport  Port=3  OutDataType=fixdt(1, 16)  OutScaling=2^0
  Add3 : Sum  Inputs=+-  OutDataType=fixdt(1, 16)  OutScaling=2^-10
  Gain6 : Gain  Gain=1/(sqrt(3))  ParameterDataType=fixdt(1, 16)  ParameterScaling=2^0  OutDataType=fixdt(1, 16)  OutScaling=2^0
  alfa : Outport  OutDataType=fixdt(1, 16)  OutScaling=2^0
  beta : Outport  Port=2  OutDataType=fixdt(1, 16)  OutScaling=2^0
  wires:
  a/1 -> alfa/1
  Gain6/1 -> beta/1
  Add3/1 -> Gain6/1
  b/1 -> Add3/1
  c/1 -> Add3/2

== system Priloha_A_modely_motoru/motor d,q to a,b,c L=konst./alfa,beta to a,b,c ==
  note: transformace alfa, beta do a, b, c
  alfa : Inport  OutDataType=fixdt(1, 16)  OutScaling=2^0
  beta : Inport  Port=2  OutDataType=fixdt(1, 16)  OutScaling=2^0
  Add1 : Sum  Inputs=--  OutDataType=fixdt(1, 16)  OutScaling=2^-10
  Add5 : Sum  Inputs=-+  OutDataType=fixdt(1, 16)  OutScaling=2^-10
  Gain1 : Gain  Gain=1/2  ParameterDataType=fixdt(1, 16)  ParameterScaling=2^0  OutDataType=fixdt(1, 16)  OutScaling=2^0
  Gain2 : Gain  Gain=sqrt(3)/2  ParameterDataType=fixdt(1, 16)  ParameterScaling=2^0  OutDataType=fixdt(1, 16)  OutScaling=2^0
  a : Outport  OutDataType=fixdt(1, 16)  OutScaling=2^0
  b : Outport  Port=2  OutDataType=fixdt(1, 16)  OutScaling=2^0
  c : Outport  Port=3  OutDataType=fixdt(1, 16)  OutScaling=2^0
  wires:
  alfa/1 -> a/1, Gain1/1
  Gain1/1 -> Add5/1, Add1/1
  Add5/1 -> b/1
  beta/1 -> Gain2/1
  Add1/1 -> c/1
  Gain2/1 -> Add5/2, Add1/2

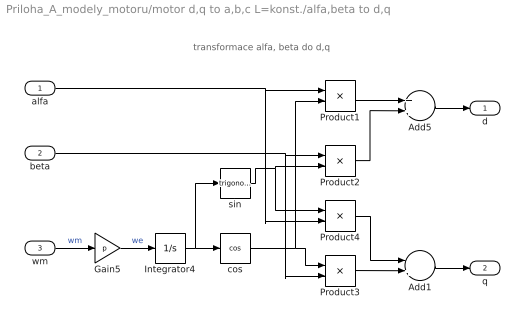
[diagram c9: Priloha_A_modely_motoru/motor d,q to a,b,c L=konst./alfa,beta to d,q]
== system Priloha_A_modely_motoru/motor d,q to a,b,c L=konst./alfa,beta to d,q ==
  note: transformace alfa, beta do d,q
  alfa : Inport  OutDataType=fixdt(1, 16)  OutScaling=2^0
  beta : Inport  Port=2  OutDataType=fixdt(1, 16)  OutScaling=2^0
  wm : Inport  Port=3  OutDataType=fixdt(1, 16)  OutScaling=2^0
  Add1 : Sum  Inputs=-+  OutDataType=fixdt(1, 16)  OutScaling=2^-10
  Add5 : Sum  OutDataType=fixdt(1, 16)  OutScaling=2^-10
  Gain5 : Gain  Gain=p  ParameterDataType=fixdt(1, 16)  ParameterScaling=2^0  OutDataType=fixdt(1, 16)  OutScaling=2^0
  Integrator4 : Integrator
  Product{1..4} (4 alike) : Product  OutDataType=fixdt(1, 16)  OutScaling=2^0
  cos : Trigonometry  Operator=cos  OutputSignalType=real
  sin : Trigonometry  OutputSignalType=real
  d : Outport  OutDataType=fixdt(1, 16)  OutScaling=2^0
  q : Outport  Port=2  OutDataType=fixdt(1, 16)  OutScaling=2^0
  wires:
  cos/1 -> Product1/2, Product3/1
  sin/1 -> Product4/1, Product2/2
  Integrator4/1 -> sin/1, cos/1
  Gain5/1 -> Integrator4/1  "we"
  wm/1 -> Gain5/1  "wm"
  Add1/1 -> q/1
  Product2/1 -> Add5/2
  beta/1 -> Product3/2, Product2/1
  alfa/1 -> Product4/2, Product1/1
  Product1/1 -> Add5/1
  Add5/1 -> d/1
  Product4/1 -> Add1/1
  Product3/1 -> Add1/2

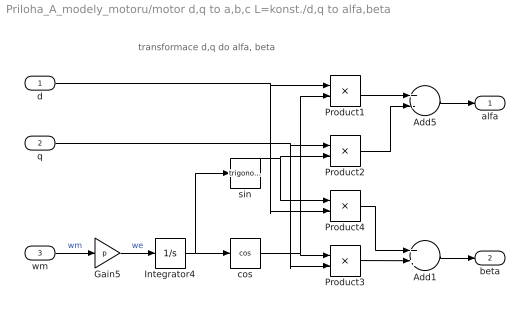
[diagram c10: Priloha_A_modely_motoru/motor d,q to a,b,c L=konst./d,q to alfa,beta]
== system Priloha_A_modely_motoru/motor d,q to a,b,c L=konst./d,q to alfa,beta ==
  note: transformace d,q do alfa, beta
  d : Inport  OutDataType=fixdt(1, 16)  OutScaling=2^0
  q : Inport  Port=2  OutDataType=fixdt(1, 16)  OutScaling=2^0
  wm : Inport  Port=3  OutDataType=fixdt(1, 16)  OutScaling=2^0
  Add1 : Sum  OutDataType=fixdt(1, 16)  OutScaling=2^-10
  Add5 : Sum  Inputs=+-  OutDataType=fixdt(1, 16)  OutScaling=2^-10
  Gain5 : Gain  Gain=p  ParameterDataType=fixdt(1, 16)  ParameterScaling=2^0  OutDataType=fixdt(1, 16)  OutScaling=2^0
  Integrator4 : Integrator
  Product{1..4} (4 alike) : Product  OutDataType=fixdt(1, 16)  OutScaling=2^0
  cos : Trigonometry  Operator=cos
  sin : Trigonometry
  alfa : Outport  OutDataType=fixdt(1, 16)  OutScaling=2^0
  beta : Outport  Port=2  OutDataType=fixdt(1, 16)  OutScaling=2^0
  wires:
  Add5/1 -> alfa/1
  Product1/1 -> Add5/1
  d/1 -> Product4/2, Product1/1
  q/1 -> Product3/2, Product2/1
  Product2/1 -> Add5/2
  Add1/1 -> beta/1
  wm/1 -> Gain5/1  "wm"
  Gain5/1 -> Integrator4/1  "we"
  Integrator4/1 -> sin/1, cos/1
  sin/1 -> Product4/1, Product2/2
  cos/1 -> Product1/2, Product3/1
  Product4/1 -> Add1/1
  Product3/1 -> Add1/2

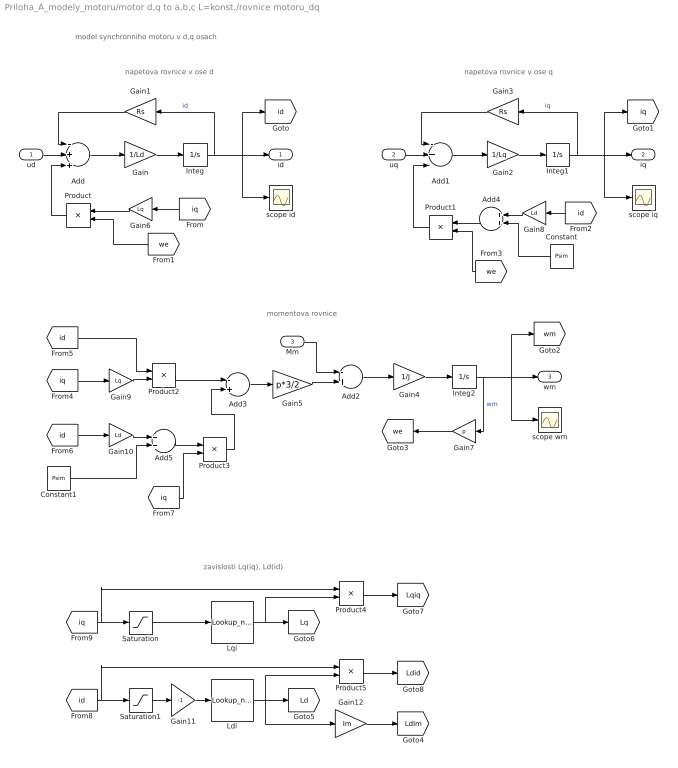
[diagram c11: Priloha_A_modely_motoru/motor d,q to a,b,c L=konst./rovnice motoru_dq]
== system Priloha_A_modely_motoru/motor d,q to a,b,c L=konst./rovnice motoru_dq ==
  note: model synchronniho motoru v d,q osach
  note: napetova rovnice v ose d
  note: napetova rovnice v ose q
  note: momentova rovnice
  note: zavislosti Lq(iq), Ld(id)
  ud : Inport  OutDataType=fixdt(1, 16)  OutScaling=2^0
  uq : Inport  Port=2  OutDataType=fixdt(1, 16)  OutScaling=2^0
  Mm : Inport  Port=3  OutDataType=fixdt(1, 16)  OutScaling=2^0
  Add : Sum  Inputs=-++  OutDataType=fixdt(1, 16)  OutScaling=2^-10
  Add1 : Sum  Inputs=-+-  OutDataType=fixdt(1, 16)  OutScaling=2^-10
  Add2 : Sum  Inputs=-+  OutDataType=fixdt(1, 16)  OutScaling=2^-10
  Add3 : Sum  Inputs=-+  OutDataType=fixdt(1, 16)  OutScaling=2^-10
  Add4 : Sum  OutDataType=fixdt(1, 16)  OutScaling=2^-10
  Add5 : Sum  OutDataType=fixdt(1, 16)  OutScaling=2^-10
  Constant : Constant  Value=Psim  OutDataType=fixdt(1, 16)  OutScaling=2^0
  Constant1 : Constant  Value=Psim  OutDataType=fixdt(1, 16)  OutScaling=2^0
  Gain : Gain  Gain=1/Ld  ParameterDataType=fixdt(1, 16)  ParameterScaling=2^0  OutDataType=fixdt(1, 16)  OutScaling=2^0
  Gain1 : Gain  Gain=Rs  ParameterDataType=fixdt(1, 16)  ParameterScaling=2^0  OutDataType=fixdt(1, 16)  OutScaling=2^0
  Gain10 : Gain  Gain=Ld  ParameterDataType=fixdt(1, 16)  ParameterScaling=2^0  OutDataType=fixdt(1, 16)  OutScaling=2^0
  Gain11 : Gain  Gain=-1  ParameterDataType=fixdt(1, 16)  ParameterScaling=2^0  OutDataType=fixdt(1, 16)  OutScaling=2^0
  Gain12 : Gain  Gain=Im  ParameterDataType=fixdt(1, 16)  ParameterScaling=2^0  OutDataType=fixdt(1, 16)  OutScaling=2^0
  Gain2 : Gain  Gain=1/Lq  ParameterDataType=fixdt(1, 16)  ParameterScaling=2^0  OutDataType=fixdt(1, 16)  OutScaling=2^0
  Gain3 : Gain  Gain=Rs  ParameterDataType=fixdt(1, 16)  ParameterScaling=2^0  OutDataType=fixdt(1, 16)  OutScaling=2^0
  Gain4 : Gain  Gain=1/J  ParameterDataType=fixdt(1, 16)  ParameterScaling=2^0  OutDataType=fixdt(1, 16)  OutScaling=2^0
  Gain5 : Gain  Gain=p*3/2  ParameterDataType=fixdt(1, 16)  ParameterScaling=2^0  OutDataType=fixdt(1, 16)  OutScaling=2^0
  Gain6 : Gain  Gain=Lq  ParameterDataType=fixdt(1, 16)  ParameterScaling=2^0  OutDataType=fixdt(1, 16)  OutScaling=2^0
  Gain7 : Gain  Gain=p  ParameterDataType=fixdt(1, 16)  ParameterScaling=2^0  OutDataType=fixdt(1, 16)  OutScaling=2^0
  Gain8 : Gain  Gain=Ld  ParameterDataType=fixdt(1, 16)  ParameterScaling=2^0  OutDataType=fixdt(1, 16)  OutScaling=2^0
  Gain9 : Gain  Gain=Lq  ParameterDataType=fixdt(1, 16)  ParameterScaling=2^0  OutDataType=fixdt(1, 16)  OutScaling=2^0
  Integ : Integrator
  Integ1 : Integrator
  Integ2 : Integrator
  Ldi : Lookup_n-D  NumberOfTableDimensions=1  BreakpointsForDimension1=[ILi]  Table=[Ldi]
  Lqi : Lookup_n-D  NumberOfTableDimensions=1  BreakpointsForDimension1=[ILi]  Table=[Lqi]
  Product{,1..5} (6 alike) : Product  OutDataType=fixdt(1, 16)  OutScaling=2^0
  Saturation : Saturate  UpperLimit=Imax  LowerLimit=ILi(1)  OutDataType=fixdt(1, 16)  OutScaling=2^0
  Saturation1 : Saturate  UpperLimit=ILi(1)  LowerLimit=-Imax  OutDataType=fixdt(1, 16)  OutScaling=2^0
  scope id : Scope
  scope iq : Scope
  scope wm : Scope
  id : Outport  OutDataType=fixdt(1, 16)  OutScaling=2^0
  iq : Outport  Port=2  OutDataType=fixdt(1, 16)  OutScaling=2^0
  wm : Outport  Port=3  OutDataType=fixdt(1, 16)  OutScaling=2^0
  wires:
  Integ/1 -> id/1, scope id/1, [id], Gain1/1  "id"
  Gain/1 -> Integ/1
  Add/1 -> Gain/1
  Gain1/1 -> Add/1
  ud/1 -> Add/2
  Integ1/1 -> Gain3/1, scope iq/1, iq/1, [iq]  "iq"
  Gain2/1 -> Integ1/1
  Add1/1 -> Gain2/1
  Gain3/1 -> Add1/1
  uq/1 -> Add1/2
  Integ2/1 -> wm/1, scope wm/1, [wm], Gain7/1  "wm"
  Gain4/1 -> Integ2/1
  Add2/1 -> Gain4/1
  Gain5/1 -> Add2/2
  Mm/1 -> Add2/1
  Add3/1 -> Gain5/1
  [iq] -> Gain6/1
  Gain6/1 -> Product/1
  Gain7/1 -> [we]
  [id] -> Gain8/1
  Gain8/1 -> Add4/1
  Add4/1 -> Product1/1
  [iq] -> Gain9/1
  [id] -> Product2/1
  Gain9/1 -> Product2/2
  Product2/1 -> Add3/1
  [id] -> Gain10/1
  Gain10/1 -> Add5/1
  Add5/1 -> Product3/1
  Constant1/1 -> Add5/2
  [iq] -> Product3/2
  Product3/1 -> Add3/2
  Product1/1 -> Add1/3
  [we] -> Product1/2
  Product/1 -> Add/3
  Constant/1 -> Add4/2
  [we] -> Product/2
  Gain12/1 -> [LdIm]
  Saturation/1 -> Lqi/1
  Saturation1/1 -> Gain11/1
  [iq] -> Saturation/1, Product4/1
  Lqi/1 -> [Lq], Product4/2
  [id] -> Saturation1/1, Product5/1
  Ldi/1 -> Gain12/1, [Ld], Product5/2
  Product4/1 -> [Lqiq]
  Product5/1 -> [Ldid]
  Gain11/1 -> Ldi/1
